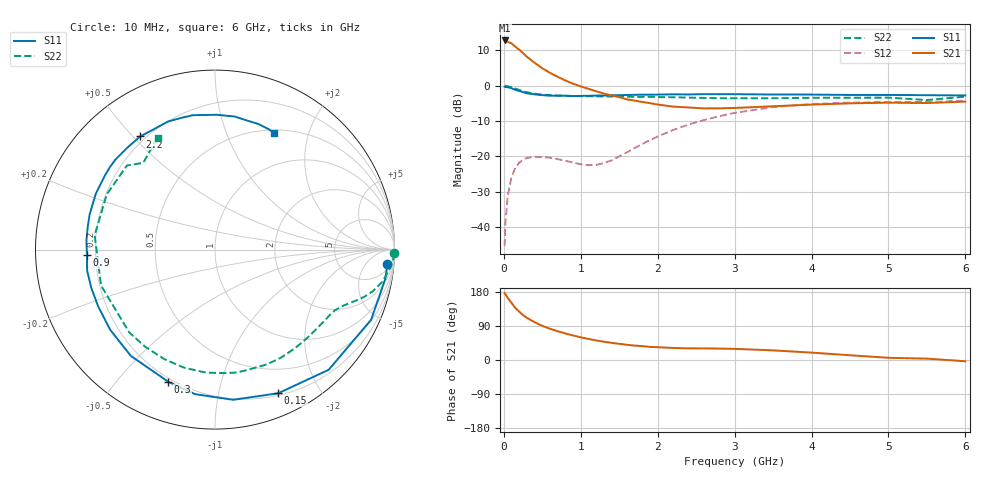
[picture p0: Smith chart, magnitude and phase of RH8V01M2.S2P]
! SIEMENS Small Signal Semiconductors
! BFR106
! Si NPN RF Bipolar Junction Transistor in SOT23
! VCE = 8 V  IC = 1.2 mA
! Common Emitter S-Parameters:  August  1996
# GHz  S  MA  R  50
!  f  S11  S21  S12  S22
! GHz  MAG  ANG  MAG  ANG  MAG  ANG  MAG  ANG
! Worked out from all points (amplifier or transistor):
!   36 points, 10 MHz to 6 GHz, reference 50 ohm
!   highest |S21| = 12.8 dB at 10 MHz (marker M1)
!   |S21| within 3 dB of that: start of sweep to 219.6 MHz
!   unconditionally stable (mu >= 1): 850.3 MHz to 1.827 GHz; 3.434 GHz to end of sweep
!   at 250 MHz: K = 0.26, MSG = 15.0 dB, |S12| = -20.9 dB
!   at 1.4 GHz: K = 1.34, MAG = 5.7 dB, |S12| = -21.1 dB
!   at 6 GHz: K = 1.02, MAG = -1.0 dB, |S12| = -4.2 dB
!   S11 on the Smith chart (normalised r, x): 10 MHz: 9, -20; 150 MHz: 0.22, -1.51; 300 MHz: 0.18, -0.69; 900 MHz: 0.17, -0.02; 2.2 GHz: 0.18, +0.52; 6 GHz: 0.54, +1.49
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0.01  0.9642 -4.8  4.362 176.3  0.0054 89.6  0.9999 -1.2
0.02  0.9631 -9.7  4.334 173.9  0.0113 82.3  0.9972 -2.4
0.05  0.9535 -24.2  4.2 164.0  0.0276 76.2  0.983 -5.8
0.1  0.9217 -46.6  3.951 150.7  0.0512 64.4  0.9496 -10.9
0.15  0.8744 -66.3  3.56 137.3  0.0695 53.9  0.9093 -14.8
0.2  0.8429 -83.1  3.229 127.5  0.0817 46.3  0.8715 -17.6
0.25  0.813 -97.9  2.881 118.2  0.0901 39.3  0.835 -19.9
0.3  0.7808 -109.5  2.562 111.3  0.0951 34.8  0.8092 -21.5
0.4  0.7554 -128.3  2.109 99.8  0.099 27.4  0.7719 -24.3
0.5  0.7353 -142.5  1.762 90.1  0.0985 23.3  0.7479 -27.0
0.7  0.7216 -162.9  1.336 75.9  0.0917 20.8  0.7275 -33.1
0.9  0.714 -177.6  1.068 64.7  0.0822 25.9  0.7155 -39.4
1.1  0.7204 169.7  0.904 55.5  0.0753 38.2  0.7094 -46.8
1.6  0.7396 146.0  0.641 40.1  0.1144 74.2  0.7004 -66.5
2.2  0.7559 123.5  0.507 31.8  0.2364 76.5  0.6874 -94.1
2.8  0.7576 104.6  0.479 30.1  0.3707 63.2  0.6668 -125.7
3.5  0.7514 89.3  0.512 25.4  0.4994 44.6  0.6657 -162.5
4  0.7495 81.6  0.541 19.5  0.5524 31.8  0.6752 173.2
4.5  0.7408 75.8  0.564 12.5  0.5774 20.6  0.677 153.0
5  0.7405 71.0  0.576 5.8  0.5884 11.6  0.6784 136.3
5.5  0.7346 65.9  0.569 3.6  0.586 7.2  0.6275 129.6
6  0.7287 63.1  0.596 -3.3  0.6165 -1.0  0.7008 117.2
